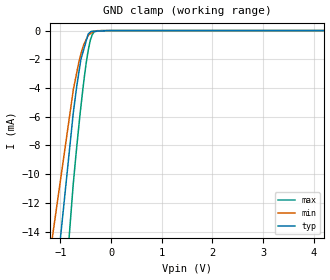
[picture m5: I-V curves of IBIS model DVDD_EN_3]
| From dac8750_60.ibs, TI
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|   DVDD_EN Models
[Model] DVDD_EN_3  |3V digital input
Model_type   Input
Vinl = 0.8
Vinh = 2
|   typ   min   max
|   (nom PVT)   (Fast PVT)   (slow PVT)
C_comp   1.578E-12   1.578E-12   1.578E-12
| Where   nom PVT is  Nominal Process, 3.0V, 36C
|   Fast PVT is Strong Process, 3.3V, -40C
|   Slow PVT is Weak Process, 2,7V, 134C
|C_comp - from L-C Tank method, L = 1nH, peak frequency
[Voltage Range]   3   2.7   3.3
|Operating Temperature   27   125   -40
|Junction Temperature
[Temperature Range]   36   134   -40
[Power Clamp Reference]   3   2.7   3.3
[GND Clamp Reference]   0   0   0
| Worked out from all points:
|   GND clamp passes 1 mA (typ) near -0.51 V on its own axis
[GND Clamp]
|   Voltage   I(typ)   I(min)   I(max)
-3V       -164.2mA   -139.3mA   -232.4mA
-1.274V   -23.9mA    -17.27mA   -34.89mA
-747.2mV  -5.775mA   -4.171mA   -10.7mA
-675.9mV  -3.838mA   -2.896mA   -8.035mA
-595.2mV  -2.001mA   -1.63mA    -5.287mA
-536.9mV  -1.287mA   -961.3uA   -3.506mA
-485.3mV  -654.8uA   -587.8uA   -2.131mA
-452.3mV  -250.2uA   -354.1uA   -1.401mA
-393.5mV  -63.15uA   -185uA     -506.3uA
-326.2mV  -40.88uA   -32.91uA   -77.31uA
-186.2mV  -22.76uA   -3.515uA   -276.8nA
5.991V    0A         0A         0A
[POWER Clamp]
|   SCR cell for ESD function. Effects occurr above VDD x 2
|   Voltage   I(typ)   I(min)   I(max)
-3V       0A         0A         0A
0V        0A         0A         0A
6V        0A         0A         0A
